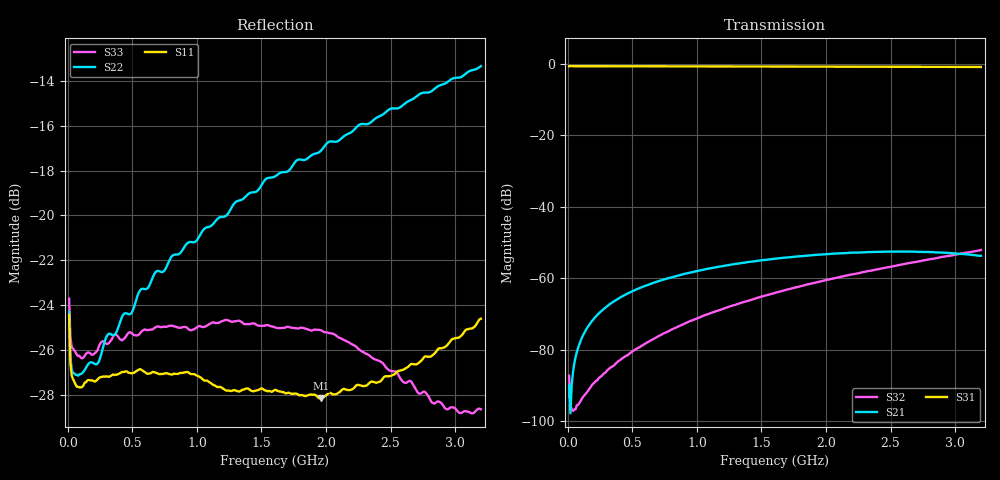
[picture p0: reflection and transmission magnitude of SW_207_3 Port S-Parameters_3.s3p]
! Created _Nov-02-2022_09-58-32
! Type : General
! Retest Level : 0
! Program : FASTESt Rev. 859
! DUT_TempC = 25.0
! Set_V1_Supply_V = 0.0
! V1_Supply_V = -0.0006
! V1_Supply_I = -4e-06
! Set_V2_Supply_V = 3.0
! V2_Supply_V = 3.0003
! V2_Supply_I = -4e-06
! RunID = 3
! SN = 2
! Comment = SW-207_SB2_RFc-RF2_room
! Input_Power = 5.0
! Measurement_Comment = None
! Freq	S11db	S11deg	S12db	S12deg	S13db	S13deg	S21db	S21deg	S22db	S22deg	S23db	S23deg	S31db	S31deg	S32db	S32deg	S33db	S33deg
# Hz S dB R 50
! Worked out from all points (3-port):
!   320 points, 10 MHz to 3.2 GHz, reference 50 ohm
!   strongest paths, dB at 10 MHz, 810 MHz, 1.61 GHz, 2.41 GHz, 3.2 GHz:
!     S31: -0.6, -0.6, -0.7, -0.7, -0.8
!     S21: -90.1, -59.6, -54.5, -52.6, -53.7
!     S32: -87.3, -74.2, -64.0, -57.4, -52.1
!   lowest |S11| = -28.2 dB at 1.96 GHz (marker M1), VSWR 1.08, Z = 46.5 + j1.48 ohm
!   |S11| at or under -10 dB: start of sweep to end of sweep
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1e7  -24.42 -43.1  -89.88 -122.5  -0.59 1.3
     -90.05 -123.6  -24.30 -38.4  -87.38 -113.0
     -0.59 1.3  -87.29 -113.8  -23.71 -40.0
7e7  -27.64 -14.3  -80.68 79.7  -0.60 -6.0
     -80.63 79.6  -27.11 -5.3  -95.59 -96.0
     -0.60 -6.0  -95.52 -92.9  -26.21 -12.8
1.8e8  -27.36 -14.5  -72.30 72.6  -0.61 -15.7
       -72.27 72.7  -26.54 4.4  -90.04 -124.0
       -0.61 -15.7  -90.32 -124.4  -26.18 -14.0
3.5e8  -27.09 -22.6  -66.62 59.6  -0.61 -30.5
       -66.59 59.6  -25.34 4.3  -84.48 -154.7
       -0.61 -30.5  -84.55 -155.0  -25.40 -24.0
8.5e8  -27.07 -69.7  -59.27 19.9  -0.63 -73.5
       -59.26 20.1  -21.74 -14.8  -73.53 143.2
       -0.63 -73.5  -73.59 143.1  -24.99 -69.7
1.21e9  -27.75 -110.5  -56.49 -8.7  -0.65 -104.4
        -56.49 -8.8  -20.06 -40.0  -68.40 107.9
        -0.64 -104.4  -68.43 107.9  -24.68 -107.0
1.61e9  -27.77 -160.0  -54.53 -40.8  -0.67 -138.7
        -54.48 -40.7  -18.24 -71.6  -63.98 74.1
        -0.67 -138.7  -64.01 74.1  -24.99 -149.5
1.96e9  -28.15 156.0  -53.36 -69.1  -0.70 -168.7
        -53.33 -69.1  -17.12 -102.2  -60.84 45.9
        -0.69 -168.7  -60.85 46.0  -25.12 175.3
2.5e9  -27.15 96.0  -52.53 -112.7  -0.74 145.0
       -52.53 -112.9  -15.25 -149.6  -56.75 5.2
       -0.74 145.0  -56.77 5.1  -26.93 119.5
3.2e9  -24.60 21.4  -53.70 -167.0  -0.82 84.8
       -53.69 -167.0  -13.34 145.4  -52.07 -45.0
       -0.81 84.7  -52.07 -44.9  -28.64 24.1
